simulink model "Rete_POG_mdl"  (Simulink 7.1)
settings: Solver=ode45  StartTime=0.0  StopTime=10.0  RelTol=1e-3
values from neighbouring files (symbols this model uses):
  C1 = 0.1*F    (= 0.1)    [Rete_POG.m]
  C2 = 0.3*F    (= 0.3)    [Rete_POG.m]
  L = 0.2*H    (= 0.2)    [Rete_POG.m]
  Phi_0 = 10*L    (= 2)    [Rete_POG.m]
  Q1_0 = 30*C1    (= 3)    [Rete_POG.m]
  Q2_0 = 30*C2    (= 9)    [Rete_POG.m]
  R1 = 10*ohm    (= 10)    [Rete_POG.m]
  R2 = 10*ohm    (= 10)    [Rete_POG.m]
  Tc = Tfin/2000    (= 0.00025)    [Rete_POG.m]

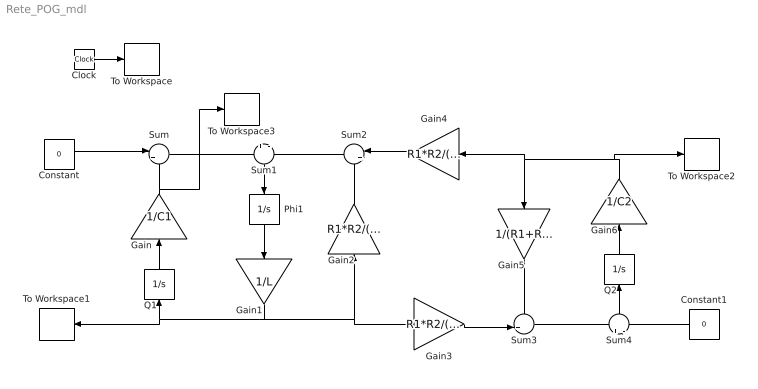
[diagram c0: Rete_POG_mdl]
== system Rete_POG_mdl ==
  Clock : Clock
  Constant : Constant  Value=0  OutDataType=sfix(16)  OutScaling=2^0
  Constant1 : Constant  Orientation=left  Value=0  OutDataType=sfix(16)  OutScaling=2^0
  Gain : Gain  Orientation=up  Gain=1/C1  ParameterDataType=sfix(16)  ParameterScaling=2^0  OutDataType=sfix(16)  OutScaling=2^0
  Gain1 : Gain  Orientation=down  Gain=1/L  ParameterDataType=sfix(16)  ParameterScaling=2^0  OutDataType=sfix(16)  OutScaling=2^0
  Gain2 : Gain  Orientation=up  Gain=R1*R2/(R1+R2)  ParameterDataType=sfix(16)  ParameterScaling=2^0  OutDataType=sfix(16)  OutScaling=2^0
  Gain3 : Gain  Gain=R1*R2/(R1+R2)  ParameterDataType=sfix(16)  ParameterScaling=2^0  OutDataType=sfix(16)  OutScaling=2^0
  Gain4 : Gain  Orientation=left  Gain=R1*R2/(R1+R2)  ParameterDataType=sfix(16)  ParameterScaling=2^0  OutDataType=sfix(16)  OutScaling=2^0
  Gain5 : Gain  Orientation=down  Gain=1/(R1+R2)  ParameterDataType=sfix(16)  ParameterScaling=2^0  OutDataType=sfix(16)  OutScaling=2^0
  Gain6 : Gain  Orientation=up  Gain=1/C2  ParameterDataType=sfix(16)  ParameterScaling=2^0  OutDataType=sfix(16)  OutScaling=2^0
  Phi1 : Integrator  Orientation=down  InitialCondition=Phi_0
  Q1 : Integrator  Orientation=up  InitialCondition=Q1_0
  Q2 : Integrator  Orientation=up  InitialCondition=Q2_0
  Sum : Sum  Inputs=|+-  OutDataType=sfix(16)  OutScaling=2^0
  Sum1 : Sum  Orientation=down  Inputs=+|-  OutDataType=sfix(16)  OutScaling=2^0
  Sum2 : Sum  Orientation=left  Inputs=|++  OutDataType=sfix(16)  OutScaling=2^0
  Sum3 : Sum  Inputs=-+|  OutDataType=sfix(16)  OutScaling=2^0
  Sum4 : Sum  Orientation=up  Inputs=+|-  OutDataType=sfix(16)  OutScaling=2^0
  To Workspace : ToWorkspace  VariableName=t  SampleTime=Tc  SaveFormat=Array
  To Workspace1 : ToWorkspace  VariableName=IL  SampleTime=Tc  SaveFormat=Array
  To Workspace2 : ToWorkspace  VariableName=V2  SampleTime=Tc  SaveFormat=Array
  To Workspace3 : ToWorkspace  VariableName=V1  SampleTime=Tc  SaveFormat=Array
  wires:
  Clock/1 -> To Workspace/1
  Constant/1 -> Sum/1
  Q1/1 -> Gain/1
  Gain/1 -> Sum/2, To Workspace3/1
  Gain1/1 -> Q1/1, To Workspace1/1, Gain2/1, Gain3/1
  Sum/1 -> Sum1/1
  Sum1/1 -> Phi1/1
  Phi1/1 -> Gain1/1
  Gain4/1 -> Sum2/1
  Sum2/1 -> Sum1/2
  Gain2/1 -> Sum2/2
  Q2/1 -> Gain6/1
  Gain6/1 -> Gain4/1, Gain5/1, To Workspace2/1
  Gain5/1 -> Sum3/1
  Gain3/1 -> Sum3/2
  Sum3/1 -> Sum4/1
  Sum4/1 -> Q2/1
  Constant1/1 -> Sum4/2
